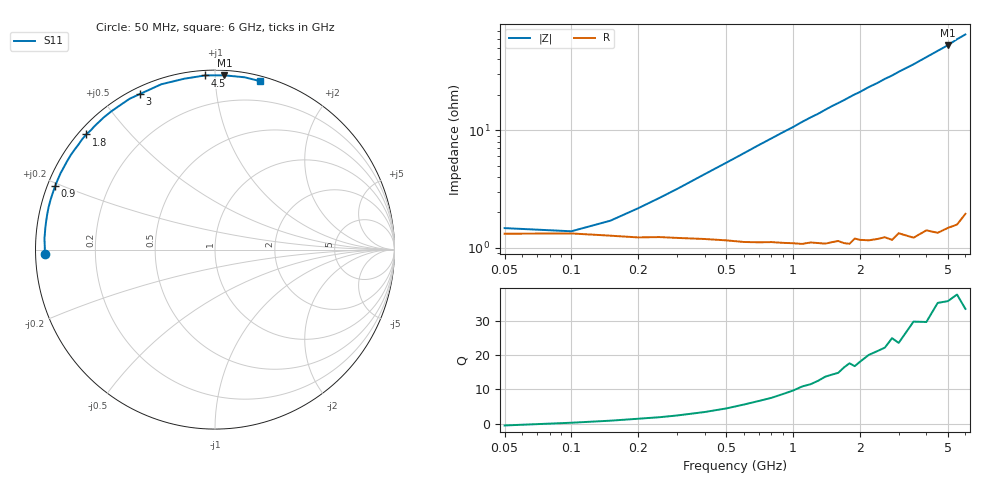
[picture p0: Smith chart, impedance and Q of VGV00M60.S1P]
! Infineon Technologies  Discrete & RF Semiconductors
! BB 831
! Si Tuning Diode in SOD323
! VR =
! S-Parameters:  July  1999
# GHz  S  MA  R  50
!  f  S11
! GHz  MAG  ANG
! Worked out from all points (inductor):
!   34 points, 50 MHz to 6 GHz, reference 50 ohm
!   read as one part to ground: L = 1.65 nH near 400 MHz
!   highest Q = 35.7 at 5 GHz (marker M1), where L = 1.68 nH
!   S11 on the Smith chart (normalised r, x): 50 MHz: 0.03, -0.01; 900 MHz: 0.02, +0.19; 1.8 GHz: 0.02, +0.38; 3 GHz: 0.03, +0.63; 4.5 GHz: 0.03, +0.95; 6 GHz: 0.04, +1.30
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0.05  0.9486 -178.5
0.1  0.9483 179.1
0.15  0.9505 177.4
0.2  0.9522 175.9
0.5  0.9552 168.2
0.6  0.9568 165.7
0.8  0.9574 160.8
0.9  0.9583 158.4
1  0.9589 156.1
1.1  0.9599 153.6
1.2  0.9591 151.3
1.3  0.96 149.2
1.5  0.9603 144.5
1.6  0.9598 142.5
1.8  0.9629 138.2
1.9  0.9595 136.1
2  0.961 134.3
2.2  0.9626 130.1
2.4  0.9627 126.6
2.6  0.9628 122.7
2.8  0.9657 119.5
3  0.9625 115.8
3.5  0.9685 108.0
4  0.9674 100.2
4.5  0.972 93.2
5  0.9724 86.9
5.5  0.9742 80.2
6  0.9716 75.0
